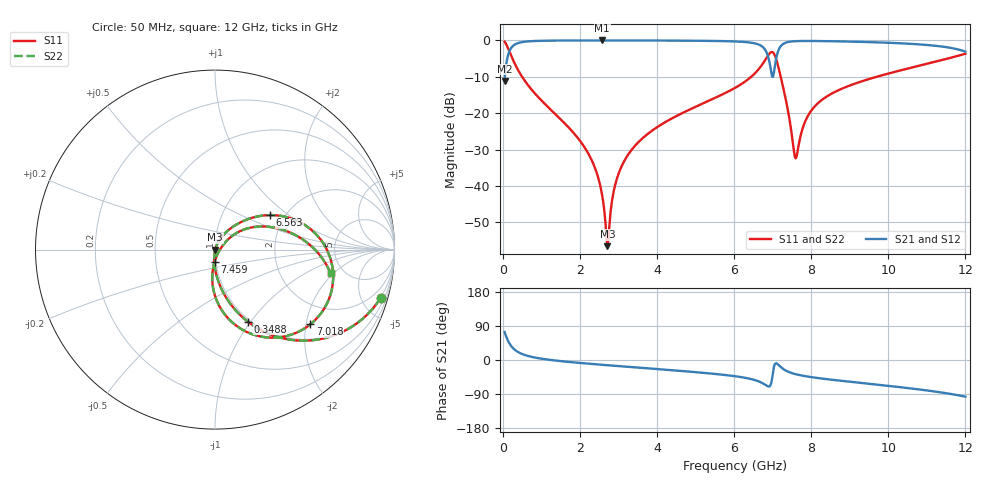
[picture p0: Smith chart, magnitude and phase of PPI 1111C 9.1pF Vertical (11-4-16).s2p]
# GHz S MA R 50
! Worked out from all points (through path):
!   1601 points, 50 MHz to 12 GHz, reference 50 ohm
!   highest |S21| = -0.01 dB at 2.582 GHz (marker M1); lowest = -11.2 dB at 50 MHz (marker M2)
!   group delay of S21, straight-line fit = 23.3 ps
!   lowest |S11| = -56.5 dB at 2.716 GHz (marker M3), VSWR 1.00, Z = 50.1 - j0.0429 ohm
!   |S11| at or under -10 dB: 504.4 MHz to 6.444 GHz (5.94 GHz wide, 171 % of centre); 7.211 GHz to 9.697 GHz (2.486 GHz wide, 29.4 % of centre)
!   |S22| runs from -56.5 to -0.3 dB; largest |S21 - S12| = 0
!   S11 on the Smith chart (normalised r, x): 50 MHz: 0.97, -6.84; 348.8 MHz: 0.97, -0.97; 6.563 GHz: 1.68, +0.74; 7.018 GHz: 1.39, -2.12; 7.459 GHz: 0.98, -0.14; 12 GHz: 3.94, -1.82
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0.05  0.9609 -16.3  0.2768 73.7  0.2768 73.7  0.9609 -16.3
0.1695  0.7141 -45.3  0.6997 44.7  0.6997 44.7  0.7141 -45.3
0.34875  0.4401 -65.6  0.8974 24.3  0.8974 24.3  0.4401 -65.6
0.916375  0.1674 -84.7  0.985 5.0  0.985 5.0  0.1674 -84.7
2.044156  0.03911 -96.3  0.9978 -8.2  0.9978 -8.2  0.03911 -96.3
2.387719  0.01804 -96.7  0.9983 -11.1  0.9983 -11.1  0.01804 -96.7
2.581906  0.007351 -91.4  0.9984 -12.7  0.9984 -12.7  0.007351 -91.4
2.716344  0.001491 -16.7  0.9983 -13.8  0.9983 -13.8  0.001491 -16.7
2.895594  0.009264 65.2  0.9982 -15.2  0.9982 -15.2  0.009264 65.2
3.09725  0.01928 68.4  0.998 -16.8  0.998 -16.8  0.01928 68.4
4.038312  0.066 64.1  0.9956 -24.1  0.9956 -24.1  0.066 64.1
6.025  0.2226 45.5  0.9676 -42.8  0.9676 -42.8  0.2226 45.5
6.56275  0.3628 32.0  0.9044 -53.6  0.9044 -53.6  0.3628 32.0
6.824156  0.5549 10.7  0.7165 -66.4  0.7165 -66.4  0.5549 10.7
6.936187  0.6737 -12.3  0.4508 -68.0  0.4508 -68.0  0.6737 -12.3
7.018344  0.6751 -38.0  0.3283 -27.3  0.3283 -27.3  0.6751 -38.0
7.197594  0.3392 -83.6  0.8143 -17.2  0.8143 -17.2  0.3392 -83.6
7.459  0.07019 -92.3  0.9618 -33.1  0.9618 -33.1  0.07019 -92.3
7.608375  0.02439 -19.1  0.9764 -37.7  0.9764 -37.7  0.02439 -19.1
8.019156  0.1114 38.6  0.9819 -45.4  0.9819 -45.4  0.1114 38.6
10.01331  0.3518 20.4  0.9278 -68.3  0.9278 -68.3  0.3518 20.4
12  0.6569 -11.6  0.7001 -96.8  0.7001 -96.8  0.6569 -11.6
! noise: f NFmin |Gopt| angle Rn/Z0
0.05  0.0003872  0.8775  2.054  0.000683
1.372  0.003737  0.673  7.436  0.002192
2.701  0.006234  0.6277  13.71  0.003096
4.031  0.008831  0.6163  19.85  0.004162
5.36  0.0132  0.6571  25.97  0.00699
6.682  0.05723  0.8901  32.78  0.1043
8.012  0.02851  0.7603  38.79  0.0215
9.341  0.02402  0.692  43.72  0.01316
10.67  0.03173  0.7365  49.16  0.02
12  0.08502  0.884  55.43  0.1248
